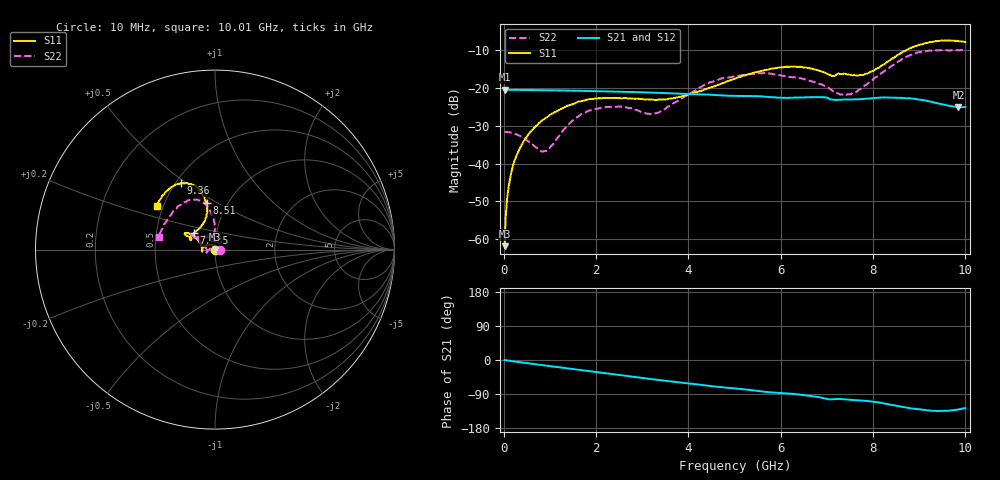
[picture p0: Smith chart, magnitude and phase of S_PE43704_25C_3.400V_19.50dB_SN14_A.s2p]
! Device ID: PE43704
! Dir: z:\PE43704\PE43704_Char_1_20130516\PE43704\AMB\3p400V\19p50dB
! Serial: 14
! Insertion: A
! Impedance: 50 ohm
! Temp: Amb
! VDD: 3.400V
! Attenuation Step: 19.50dB
! IDD: 1.139536e-01mA
#  Hz  S  RI  R  50
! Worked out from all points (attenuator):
!   401 points, 10 MHz to 10.01 GHz, reference 50 ohm
!   highest |S21| = -20.47 dB at 10 MHz (marker M1); lowest = -25.1 dB at 9.86 GHz (marker M2)
!   lowest |S11| = -61.9 dB at 10 MHz (marker M3), VSWR 1.00, Z = 50.1 + j0.0433 ohm
!   |S11| at or under -10 dB: start of sweep to 8.727 GHz
!   |S22| runs from -36.8 to -9.9 dB; largest |S21 - S12| = 0.001
!   S11 on the Smith chart (normalised r, x): 10 MHz: 1.00, +0.00; 7.485 GHz: 0.78, +0.15; 8.51 GHz: 0.80, +0.45; 9.36 GHz: 0.53, +0.48; 10.01 GHz: 0.46, +0.27
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1e7  0.000681 0.000432  0.0947 -0.000301  0.0947 -0.000308  0.0261 0.000221
8.5e7  0.000774 0.00429  0.0946 -0.00248  0.0945 -0.00245  0.0259 0.00238
1.6e8  0.000383 0.0078  0.0944 -0.00458  0.0944 -0.00451  0.0252 0.0047
2.6e8  -0.00146 0.0122  0.094 -0.00719  0.0941 -0.00721  0.0231 0.00765
4.1e8  -0.00491 0.0183  0.0933 -0.0115  0.0933 -0.0111  0.0191 0.0112
9.1e8  -0.0279 0.029  0.0902 -0.0239  0.0901 -0.0238  -0.00492 0.0138
1.685e9  -0.0654 0.0143  0.0815 -0.0417  0.0815 -0.0418  -0.0443 -0.00993
2.36e9  -0.0734 -0.00494  0.071 -0.0547  0.0711 -0.0546  -0.0508 -0.0248
3.36e9  -0.0704 -0.0019  0.0519 -0.0685  0.0521 -0.0685  -0.0474 0.00192
4.41e9  -0.0883 0.042  0.0312 -0.0757  0.0313 -0.0756  -0.0954 0.0619
5.01e9  -0.1126 0.0703  0.0203 -0.0758  0.0203 -0.0759  -0.1223 0.0737
5.96e9  -0.1609 0.0933  0.0041 -0.0745  0.00424 -0.0744  -0.1279 0.0743
6.685e9  -0.1614 0.0791  -0.00722 -0.0752  -0.00732 -0.0751  -0.1007 0.0688
7.11e9  -0.1309 0.0612  -0.0163 -0.0683  -0.0165 -0.0687  -0.0562 0.0748
7.485e9  -0.1174 0.0934  -0.018 -0.0681  -0.0179 -0.068  -0.0204 0.0804
7.835e9  -0.0749 0.1337  -0.0221 -0.0683  -0.0219 -0.0683  -0.00144 0.1086
8.36e9  -0.0437 0.2255  -0.0341 -0.0662  -0.0342 -0.0666  -0.0127 0.1849
8.51e9  -0.0467 0.2602  -0.0378 -0.0637  -0.0376 -0.0639  -0.0247 0.2138
8.935e9  -0.098 0.3452  -0.0451 -0.0551  -0.0451 -0.0549  -0.0897 0.2744
9.36e9  -0.1884 0.3709  -0.0443 -0.0454  -0.0447 -0.0452  -0.1804 0.2598
9.86e9  -0.2975 0.2903  -0.0359 -0.0424  -0.0362 -0.0422  -0.2886 0.1278
1.001e10  -0.3235 0.2439  -0.0341 -0.0448  -0.0342 -0.0447  -0.3121 0.0694
